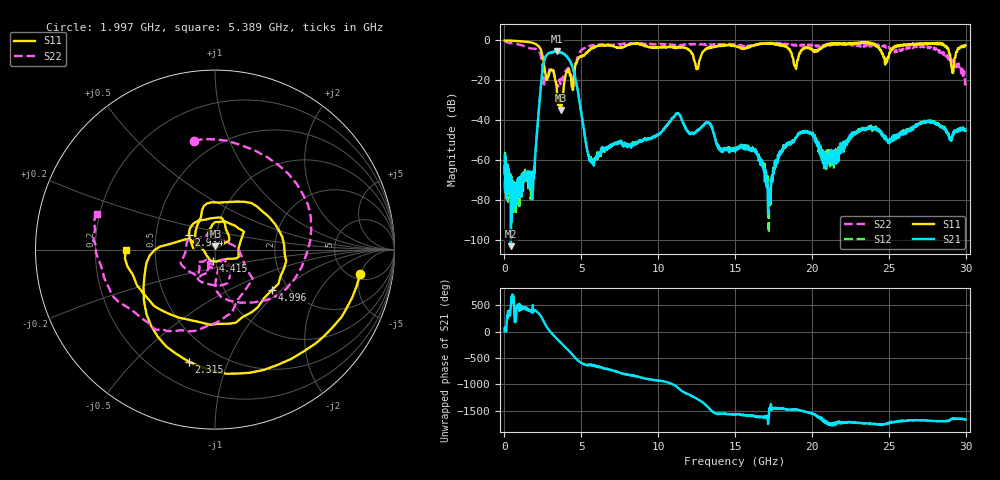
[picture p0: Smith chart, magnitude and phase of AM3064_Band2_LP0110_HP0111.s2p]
# Hz S DB R 50.0
!freq dBS11 angS11 dBS21 angS21 dBS12 angS12 dBS22 angS22
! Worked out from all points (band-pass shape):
!   1600 points, 10 MHz to 29.98 GHz, reference 50 ohm
!   highest |S21| = -5.51 dB at 3.403 GHz (marker M1); lowest = -102.9 dB at 422.4 MHz (marker M2)
!   |S21| within 3 dB of the highest: 2.652 GHz to 4.091 GHz (1.439 GHz wide, 42.7 % of centre)
!   lowest |S11| = -34.9 dB at 3.684 GHz (marker M3), VSWR 1.04, Z = 50.2 + j1.8 ohm
!   |S11| at or under -10 dB: 2.535 GHz to 4.737 GHz (2.202 GHz wide, 60.6 % of centre); 12.34 GHz to 12.68 GHz (341.7 MHz wide, 2.73 % of centre); 18.8 GHz to 19.05 GHz (251.2 MHz wide, 1.33 % of centre)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
!   |S22| runs from -23.5 to -0.3 dB; largest |S21 - S12| = 0.013
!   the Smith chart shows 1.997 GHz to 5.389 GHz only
!   S11 on the Smith chart (normalised r, x): 1.997 GHz: 5.86, -4.91; 2.315 GHz: 0.35, -0.73; 2.934 GHz: 0.74, +0.12; 4.415 GHz: 0.97, -0.13; 4.996 GHz: 1.65, -0.87; 5.389 GHz: 0.33, -0.00
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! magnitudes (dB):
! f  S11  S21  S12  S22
! 10 MHz  0.0  -62.5  -56.8  -0.3
! 422.4 MHz  -0.1  -102.9  -75.8  -1.4
! 1.791 GHz  -1.2  -72.0  -68.4  -4.1
! 1.997 GHz  -1.7  -58.1  -57.0  -4.2
! 2.315 GHz  -3.9  -27.6  -27.5  -6.5
! 2.934 GHz  -15.5  -6.3  -6.3  -14.4
! 3.403 GHz  -24.4  -5.5  -5.6  -22.5
! 3.684 GHz  -34.9  -6.1  -6.0  -20.5
! 4.415 GHz  -23.6  -13.2  -13.1  -21.4
! 4.996 GHz  -8.2  -35.9  -35.9  -5.2
! 5.015 GHz  -8.3  -37.2  -36.9  -5.0
! 5.389 GHz  -6.0  -55.4  -55.2  -3.2
! 10 GHz  -3.5  -47.0  -47.1  -1.9
! 11.27 GHz  -3.6  -36.5  -36.4  -2.6
! 15 GHz  -2.6  -54.7  -55.7  -2.0
! 16.32 GHz  -2.3  -54.3  -54.1  -2.2
! 17.18 GHz  -1.7  -80.8  -90.4  -1.6
! 18.19 GHz  -2.2  -53.3  -53.3  -1.9
! 19.99 GHz  -4.2  -46.9  -46.8  -2.2
! 21.04 GHz  -1.9  -61.6  -57.7  -2.2
! 25 GHz  -8.0  -50.7  -50.8  -3.3
! 29.98 GHz  -2.4  -45.0  -45.4  -20.3
